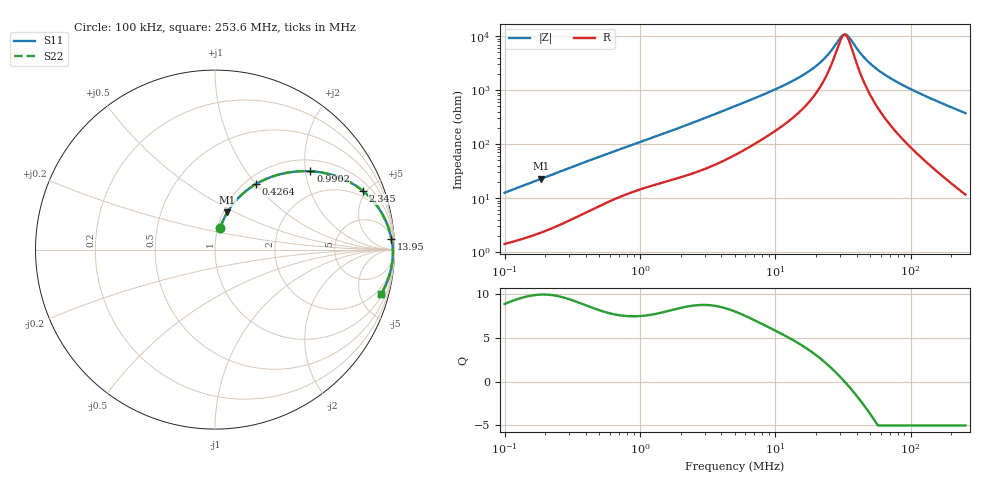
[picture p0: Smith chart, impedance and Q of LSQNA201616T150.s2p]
! LSQNA201616T150  S-PARAMETER MODEL  ( General Type )
! Model Generated by TAIYO YUDEN Corporation (http://www.ty-top.com)
! Version 2.0
! TAIYO YUDEN Control No. 100810NF25SB-FKC
! Copyright(c) 2007 TAIYO YUDEN CO.,LTD. All Rights Reserved.
! Product Description (link to TY-COMPAS)
! https://ds.yuden.co.jp/TYCOMPAS/or/detail?pn=LSQNA201616T150K&u=M
! Products Name : Inductors
! Characteristics :
!  Inductance : 15 uH , SRF(min) : 28 MHz , DC Resistance(max) : 0.91 Ohm
!  Rated Current : Saturation :210 mA , Temp Rise : 440 mA (40 degC)
!  Case Size : 2.0 x 1.6 / 0.079 x 0.063 [mm/inch] , Thickness : 1.6 / 0.063 [mm/inch]
!  (Conditions: Temperature = 25 degC , DC Bias Current/Voltage = 0A / 0V)
! External Node Assignments :
!  1  o---GGG---o  2
! GND o---------o GND
! Frequency Range : 0.1MHz  -  253.640152MHz  [ 402 STEP ]
# MHz S RI R 50
! Freq[MHz].  S11 Real  S11 Imag  S21 Real  S21 Imag  S12 Real  S12 Imag  S22 Real  S22 Imag
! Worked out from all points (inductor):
!   401 points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, 100 kHz to 253.6 MHz, reference 50 ohm
!   read as one part in series: L = 19.7 uH near 104 kHz
!   highest Q = 9.91 at 187.2 kHz (marker M1), where L = 19.4 uH
!   self-resonance near 32.4 MHz
!   S11 on the Smith chart (normalised r, x): 100 kHz: 1.03, +0.25; 426.4 kHz: 1.12, +1.00; 990.2 kHz: 1.29, +2.13; 2.345 MHz: 1.55, +4.74; 13.95 MHz: 8, +30; 253.6 MHz: 1.23, -7.50
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0.1  0.0286 0.1195  0.9714 -0.1195  0.9714 -0.1195  0.0286 0.1195
0.187214  0.0689 0.2078  0.9311 -0.2078  0.9311 -0.2078  0.0689 0.2078
0.371712  0.1889 0.339  0.8111 -0.339  0.8111 -0.339  0.1889 0.339
0.426364  0.2267 0.364  0.7733 -0.364  0.7733 -0.364  0.2267 0.364
0.656164  0.372 0.4223  0.628 -0.4223  0.628 -0.4223  0.372 0.4223
0.990225  0.5319 0.4364  0.4681 -0.4364  0.4681 -0.4364  0.5319 0.4364
1.381698  0.6597 0.414  0.3403 -0.414  0.3403 -0.414  0.6597 0.414
2.345296  0.8239 0.3272  0.1761 -0.3272  0.1761 -0.3272  0.8239 0.3272
5.03627  0.9413 0.1807  0.0587 -0.1807  0.0587 -0.1807  0.9413 0.1807
9.245617  0.973 0.0995  0.027 -0.0995  0.027 -0.0995  0.973 0.0995
13.95267  0.9828 0.0608  0.0172 -0.0608  0.0172 -0.0608  0.9828 0.0608
18.72042  0.987 0.0379  0.013 -0.0379  0.013 -0.0379  0.987 0.0379
23.68329  0.9892 0.0213  0.0108 -0.0213  0.0108 -0.0213  0.9892 0.0213
30.55478  0.9906 0.00409  0.00939 -0.00409  0.00939 -0.00409  0.9906 0.00409
33.04618  0.9909 -0.00117  0.00915 0.00117  0.00915 0.00117  0.9909 -0.00117
35.04717  0.991 -0.00513  0.00902 0.00513  0.00902 0.00513  0.991 -0.00513
41.80689  0.9911 -0.0172  0.00892 0.0172  0.00892 0.0172  0.9911 -0.0172
47.95365  0.9909 -0.0271  0.00914 0.0271  0.00914 0.0271  0.9909 -0.0271
57.20271  0.9902 -0.0405  0.00984 0.0405  0.00984 0.0405  0.9902 -0.0405
69.58603  0.9887 -0.0568  0.0113 0.0568  0.0113 0.0568  0.9887 -0.0568
120.4529  0.9785 -0.1157  0.0215 0.1157  0.0215 0.1157  0.9785 -0.1157
253.6402  0.9271 -0.245  0.0729 0.245  0.0729 0.245  0.9271 -0.245
